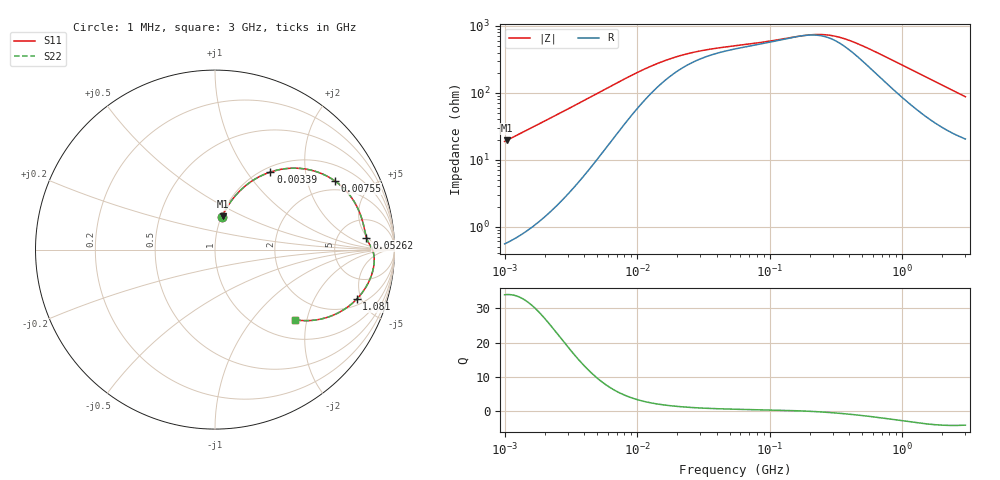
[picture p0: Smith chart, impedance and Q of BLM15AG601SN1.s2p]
! BLM15AG601SN1
# Hz S RI R 50
!Freq.(Hz) S11(Real) S11(Imag) S21(Real) S21(Imag) S12(Real) S12(Imag) S22(Real) S22(Imag)
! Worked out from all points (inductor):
!   401 points, 1 MHz to 3 GHz, reference 50 ohm
!   read as one part in series: L = 2.99 uH near 1.041 MHz
!   highest Q = 34 at 1.041 MHz (marker M1), where L = 2.99 uH
!   self-resonance near 174.8 MHz
!   S11 on the Smith chart (normalised r, x): 1 MHz: 1.01, +0.38; 3.39 MHz: 1.08, +1.30; 7.55 MHz: 1.58, +2.97; 52.62 MHz: 10, +5; 1.081 GHz: 2.50, -4.58; 3 GHz: 1.41, -1.70
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1000000  0.0389 0.1793  0.9611 -0.1793  0.9611 -0.1793  0.0389 0.1793
1040844  0.0418 0.186  0.9582 -0.186  0.9582 -0.186  0.0418 0.186
1974946  0.1311 0.3197  0.8689 -0.3197  0.8689 -0.3197  0.1311 0.3197
2613693  0.2089 0.3841  0.7911 -0.3841  0.7911 -0.3841  0.2089 0.3841
3390478  0.3084 0.4321  0.6916 -0.4321  0.6916 -0.4321  0.3084 0.4321
3823119  0.3621 0.4462  0.6379 -0.4462  0.6379 -0.4462  0.3621 0.4462
5266264  0.5157 0.4466  0.4843 -0.4466  0.4843 -0.4466  0.5157 0.4466
7550455  0.6669 0.3833  0.3331 -0.3833  0.3331 -0.3833  0.6669 0.3833
1.019448e7  0.7491 0.3053  0.2509 -0.3053  0.2509 -0.3053  0.7491 0.3053
1.461624e7  0.8007 0.2184  0.1993 -0.2184  0.1993 -0.2184  0.8007 0.2184
2.611722e7  0.8306 0.1238  0.1694 -0.1238  0.1694 -0.1238  0.8306 0.1238
5.262293e7  0.844 0.0651  0.156 -0.0651  0.156 -0.0651  0.844 0.0651
5.477226e7  0.8447 0.0629  0.1553 -0.0629  0.1553 -0.0629  0.8447 0.0629
2.094008e8  0.8818 -0.015  0.1182 0.015  0.1182 0.015  0.8818 -0.015
2.771263e8  0.8866 -0.0434  0.1134 0.0434  0.1134 0.0434  0.8866 -0.0434
3.594878e8  0.8864 -0.0755  0.1136 0.0755  0.1136 0.0755  0.8864 -0.0755
4.853736e8  0.8788 -0.1199  0.1212 0.1199  0.1212 0.1199  0.8788 -0.1199
8.005644e8  0.8388 -0.2123  0.1612 0.2123  0.1612 0.2123  0.8388 -0.2123
1.080907e9  0.7895 -0.2759  0.2105 0.2759  0.2105 0.2759  0.7895 -0.2759
1.430499e9  0.7199 -0.3332  0.2801 0.3332  0.2801 0.3332  0.7199 -0.3332
1.931433e9  0.6194 -0.3794  0.3806 0.3794  0.3806 0.3794  0.6194 -0.3794
3e9  0.4461 -0.3913  0.5539 0.3913  0.5539 0.3913  0.4461 -0.3913
